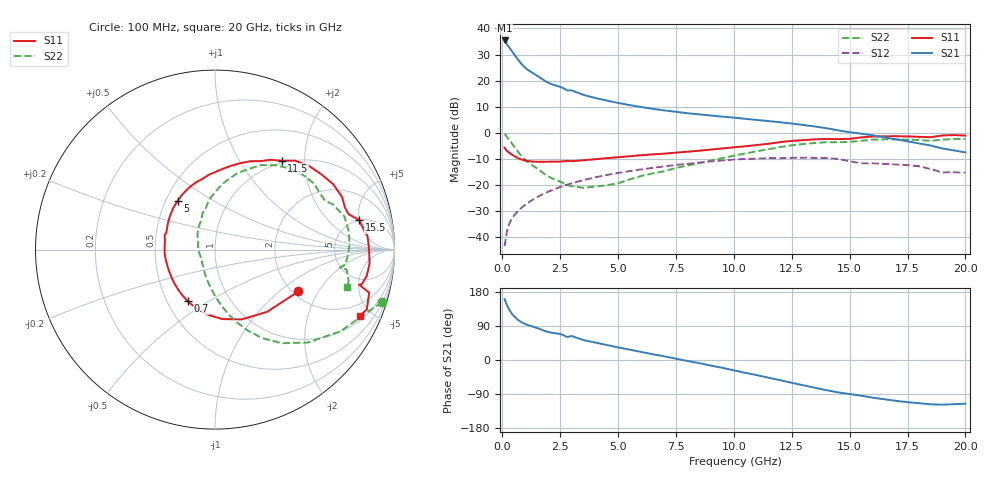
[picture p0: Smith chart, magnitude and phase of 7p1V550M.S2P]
! Infineon Technologies  Discrete & RF Semiconductors
! bfp620
! VCE =  1.5 V,  IC =  50 mA
! Common Emitter S-Parameters:  Sep 2002
# GHz  S  MA  R  50
!  f  S11  S21  S12  S22
! GHz  MAG  ANG  MAG  ANG  MAG  ANG  MAG  ANG
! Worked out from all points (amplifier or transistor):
!   59 points, 100 MHz to 20 GHz, reference 50 ohm
!   highest |S21| = 35.4 dB at 100 MHz (marker M1)
!   |S21| within 3 dB of that: start of sweep to 325 MHz
!   unconditionally stable (mu >= 1): 2.68 GHz to 2.944 GHz; 3.102 GHz to 9.851 GHz; 17.18 GHz to end of sweep
!   at 1 GHz: K = 0.85, MSG = 26.2 dB, |S12| = -27.5 dB
!   at 5.5 GHz: K = 1.04, MAG = 11.5 dB, |S12| = -14.6 dB
!   at 20 GHz: K = 1.31, MAG = 0.6 dB, |S12| = -15.3 dB
!   S11 on the Smith chart (normalised r, x): 100 MHz: 2.14, -1.37; 700 MHz: 0.63, -0.41; 5 GHz: 0.58, +0.35; 11.5 GHz: 0.96, +1.54; 15.5 GHz: 4.97, +4.99; 20 GHz: 1.22, -4.29
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0.1  0.5202 -26.6  58.71 160.7  0.0068 76.5  0.9747 -17.5
0.2  0.4521 -50.1  49.6 145.1  0.0131 71.4  0.8341 -33.1
0.3  0.4166 -68.9  43.03 132.9  0.0181 68.7  0.7306 -45.2
0.4  0.3892 -84.0  37.46 123.4  0.0223 66.7  0.6403 -54.5
0.5  0.3644 -96.9  32.49 116.0  0.026 65.3  0.5581 -62.0
0.6  0.3427 -108.1  28.15 109.9  0.0294 64.4  0.4851 -68.1
0.7  0.3251 -117.9  24.49 104.9  0.0327 63.7  0.4231 -73.3
0.8  0.3118 -126.4  21.54 100.8  0.0359 63.3  0.3725 -77.7
0.9  0.302 -133.6  19.24 97.4  0.0391 62.9  0.3325 -81.5
1.1  0.2898 -144.8  16.12 92.3  0.0456 62.4  0.277 -87.5
1.9  0.2807 -174.8  9.555 75.4  0.0721 58.2  0.1552 -109.7
2.8  0.2917 164.1  6.51 60.6  0.1021 51.0  0.0997 -138.0
3  0.2873 160.8  6.509 63.2  0.1086 49.3  0.0958 -137.4
3.5  0.2995 151.5  5.346 52.6  0.125 44.6  0.0889 -157.0
5  0.3424 127.4  3.746 33.2  0.1714 30.0  0.1086 149.3
7  0.4006 100.0  2.691 9.6  0.229 10.3  0.1851 113.9
10.5  0.554 62.8  1.859 -33.9  0.3173 -29.6  0.4031 78.6
11.5  0.6187 53.2  1.683 -46.8  0.329 -42.0  0.4875 67.2
13.5  0.7525 29.0  1.326 -73.2  0.3327 -66.0  0.6417 41.0
15.5  0.8196 11.6  0.967 -94.1  0.262 -88.2  0.7049 20.8
17  0.8649 -5.3  0.756 -107.7  0.2488 -97.7  0.7502 2.5
20  0.8893 -24.4  0.424 -115.3  0.1723 -107.6  0.7658 -15.9
